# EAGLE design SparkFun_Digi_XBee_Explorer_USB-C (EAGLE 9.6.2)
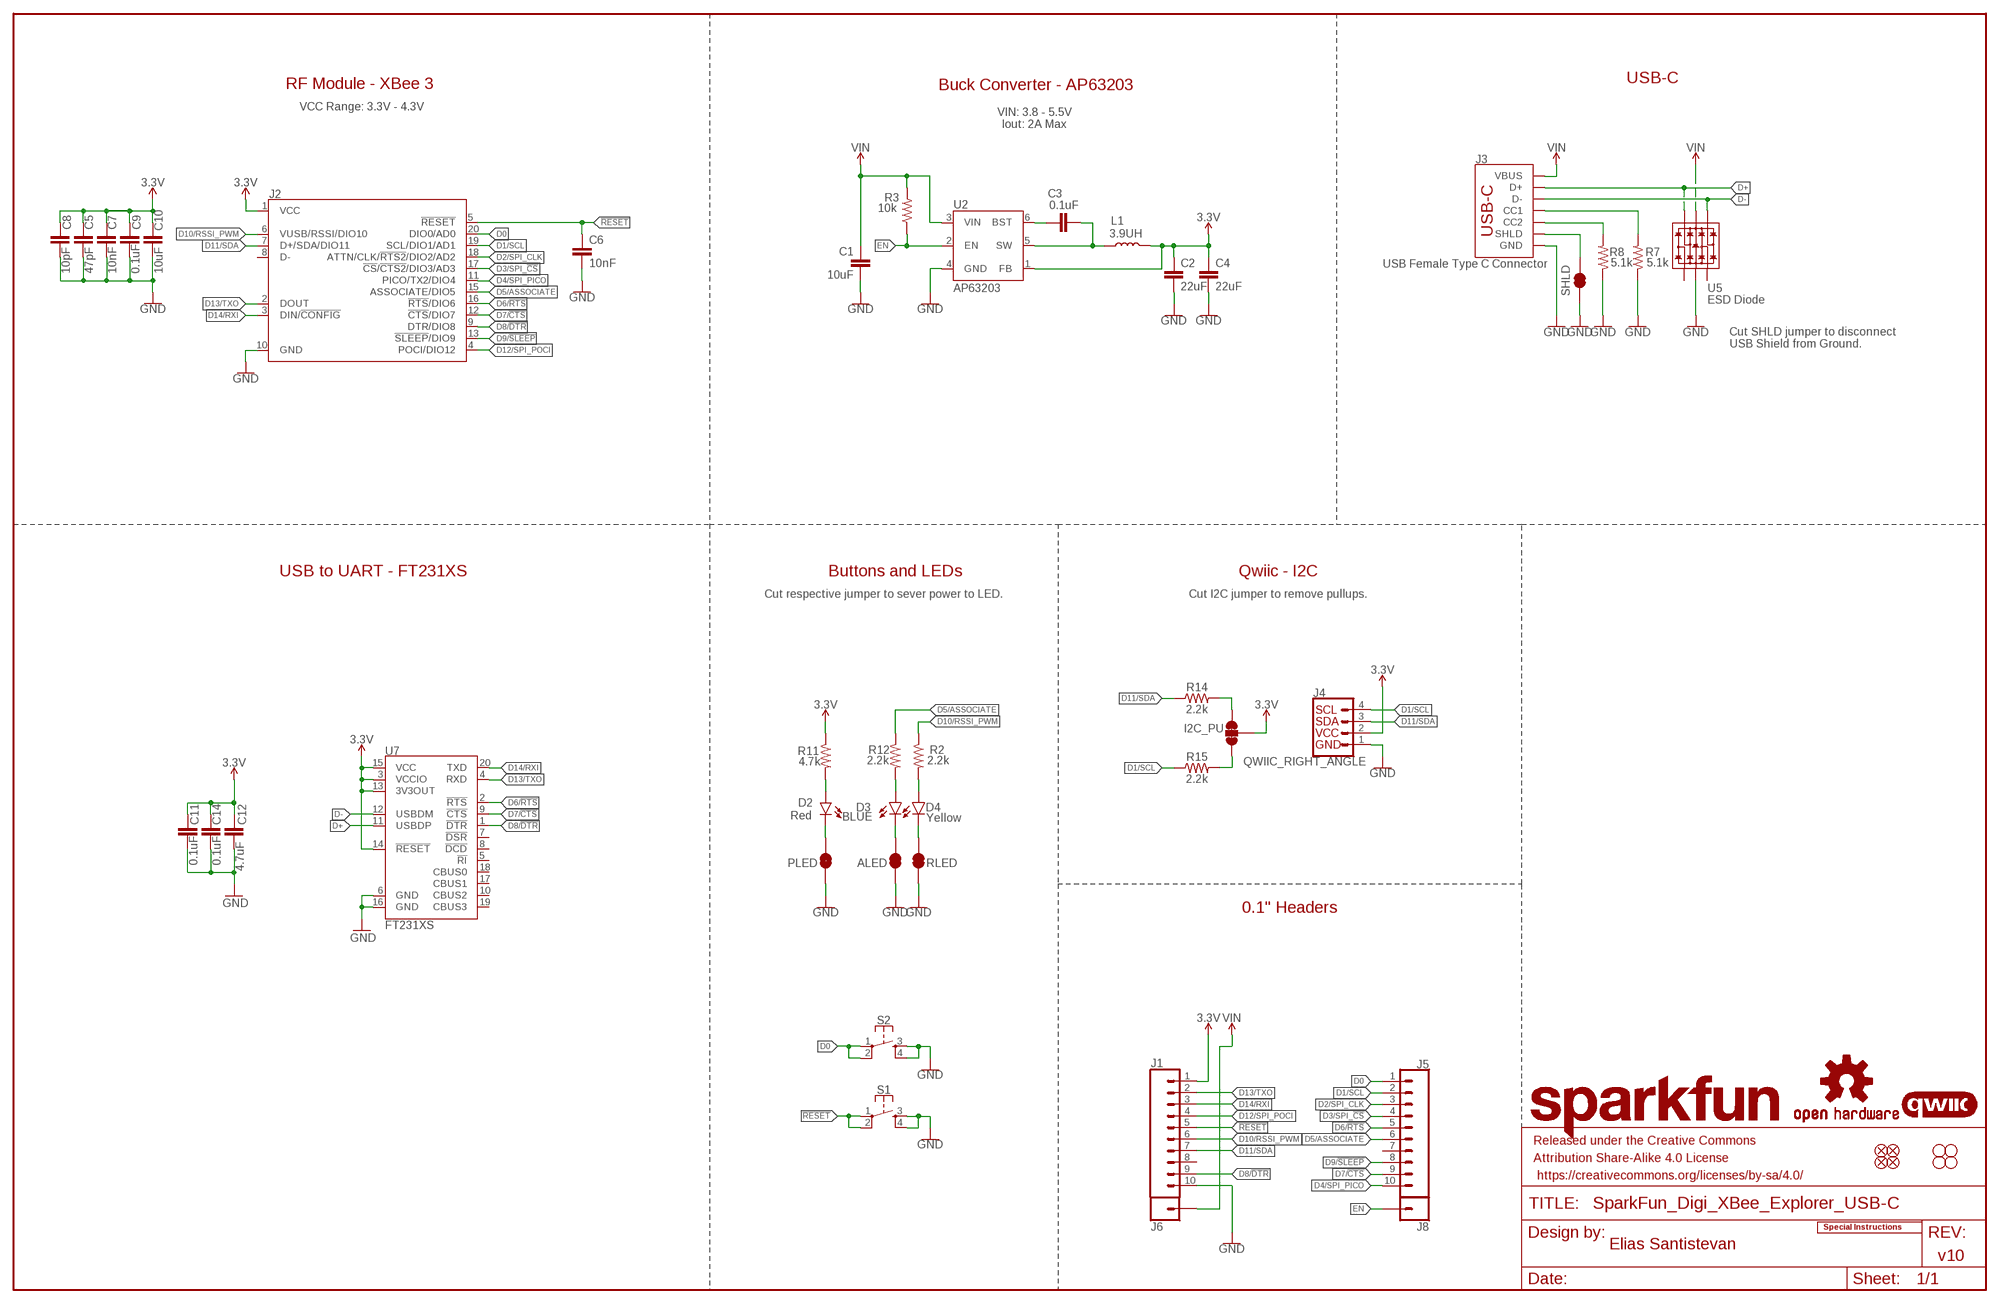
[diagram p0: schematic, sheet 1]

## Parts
ALED  JUMPER-SMT_2_NC_TRACE_SILK  [SMT-JUMPER_2_NC_TRACE_SILK]
C1  10uF  10UF-1210-50V-20%  [1210]
C2  22uF  22UF-0603-6.3V-20%  [0603]
C3  0.1uF  0.1UF-0603-25V-5%  [0603]
C4  22uF  22UF-0603-6.3V-20%  [0603]
C5  47pF  47PF-0603-50V-5%  [0603]
C6  10nF  10NF-0603-50V-10%  [0603]
C7  10nF  10NF-0603-50V-10%  [0603]
C8  10pF  10PF-0603-50V-5%  [0603]
C9  0.1uF  0.1UF-0603-25V-(+80/-20%)  [0603]
C10  10uF  10UF-0603-6.3V-20%  [0603]
C11  0.1uF  0.1UF-0603-25V-(+80/-20%)  [0603]
C12  4.7uF  4.7UF-0603-6.3V-(10%)  [0603]
C14  0.1uF  0.1UF-0603-25V-(+80/-20%)  [0603]
D2  Red  LED-RED_0603-KB  [LED-0603]
D3  BLUE  LED-BLUE0603  [LED-0603]
D4  Yellow  LED-YELLOW0603  [LED-0603]
FD1  FIDUCIAL1X2  [FIDUCIAL-1X2]
FD2  FIDUCIAL1X2  [FIDUCIAL-1X2]
FD3  FIDUCIAL1X2  [FIDUCIAL-1X2]
FD4  FIDUCIAL1X2  [FIDUCIAL-1X2]
FRAME1  FRAME-LEDGER  [CREATIVE_COMMONS]
H1  STAND-OFFTIGHT  [STAND-OFF-TIGHT]
H2  STAND-OFFTIGHT  [STAND-OFF-TIGHT]
H3  STAND-OFFTIGHT  [STAND-OFF-TIGHT]
H4  STAND-OFFTIGHT  [STAND-OFF-TIGHT]
I2C_PU  JUMPER-SMT_3_2-NC_TRACE_SILK  [SMT-JUMPER_3_2-NC_TRACE_SILK]
J1  CONN_01PTH_NO_SILK_STAND  [1X01_NO_SILK_STAND]
J2  XBEE_UPDATEXBEE_SMD  [XBEE3-SMD]
J3  USB Female Type C Connector  USB_C_4-LAYER-ISOLATED  [USB-C-16P-4LAYER-ISOLATED]
J4  QWIIC_RIGHT_ANGLE  QWIIC_CONNECTORJS-1MM  [JST04_1MM_RA]
J5  CONN_10NO_SILK_PTH_FEMALE  [1X10_NO_SILK]
J6  CONN_10NO_SILK_PTH_FEMALE  [1X10_NO_SILK]
J8  CONN_01PTH_NO_SILK_STAND  [1X01_NO_SILK_STAND]
L1  3.9UH  [INDUCTOR_3.9UH]
LOGO1  SFE_LOGO_NAME.2_INCH  [SFE_LOGO_NAME_.2]
LOGO2  OSHW-LOGOS  [OSHW-LOGO-S]
LOGO3  QWIIC_LOGO_4MM  [QWIIC_4MM]
LOGO4  SPECIAL_INSTRUCTIONS-ORDERING  [ORDERING_INSTRUCTIONS]
PLED  JUMPER-SMT_2_NC_TRACE_SILK  [SMT-JUMPER_2_NC_TRACE_SILK]
R2  2.2k  2.2KOHM-0603-1/10W-1%  [0603]
R3  10k  10KOHM-0603-1/10W-1%  [0603]
R7  5.1k  5.1KOHM5.1KOHM-0603-1/10W-1%  [0603]
R8  5.1k  5.1KOHM5.1KOHM-0603-1/10W-1%  [0603]
R11  4.7k  4.7KOHM-0603-1/10W-1%  [0603]
R12  2.2k  2.2KOHM-0603-1/10W-1%  [0603]
R14  2.2k  2.2KOHM-0603-1/10W-1%  [0603]
R15  2.2k  2.2KOHM-0603-1/10W-1%  [0603]
RLED  JUMPER-SMT_2_NC_TRACE_SILK  [SMT-JUMPER_2_NC_TRACE_SILK]
S1  MOMENTARY-SWITCH-SPST-2-SMD-5.2MM-TALL  [TACTILE_SWITCH_SMD_5.2MM]
S2  MOMENTARY-SWITCH-SPST-2-SMD-5.2MM-TALL  [TACTILE_SWITCH_SMD_5.2MM]
SHLD  JUMPER-SMT_2_NC_TRACE_SILK  [SMT-JUMPER_2_NC_TRACE_SILK]
U2  AP63203  [SOT23-6]
U5  ESD Diode  TVS_DIODE_ARRAY_DT1042-04SO-7  [SOT-23-6]
U7  FT231XS  [SSOP20_L]

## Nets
3.3V: C2.1 C4.1 C5.1 C7.1 C8.1 C9.1 C10.1 C11.1 C12.1 C14.1 I2C_PU.2 J2.1(VCC) J4.2 J6.1 L1.P$2 R11.1 U2.1(FB) U7.3(VCCIO) U7.13(3V3OUT) U7.14(!RESET) U7.15(VCC)
!RESET!: C6.1 J2.5(!RESET!) J6.5 S1.1 S1.2
D0: J2.20(DIO0/AD0) J5.1 S2.1 S2.2
D1/SCL: J2.19(SCL/DIO1/AD1) J4.4 J5.2 R15.1
D2/SPI_CLK: J2.18(ATTN/CLK/!RTS2!/DIO2/AD2) J5.3
D3/SPI_!CS!: J2.17(!CS!/!CTS2!/DIO3/AD3) J5.4
D4/SPI_PICO: J2.11(PICO/TX2/DIO4) J5.10
D5/ASSOCIATE: J2.15(ASSOCIATE/DIO5) J5.6 R12.1
D6/!RTS!: J2.16(!RTS!/DIO6) J5.5 U7.2(!RTS)
D7/!CTS!: J2.12(!CTS!/DIO7) J5.9 U7.9(!CTS)
D8/!DTR!: J2.9(DTR/DIO8) J6.9 U7.1(!DTR)
D9/!SLEEP!: J2.13(!SLEEP!/DIO9) J5.8
D10/RSSI_PWM: J2.6(VUSB/RSSI/DIO10) J6.6 R2.1
D11/SDA: J2.7(D+/SDA/DIO11) J4.3 J6.7 R14.1
D12/SPI_POCI: J2.4(POCI/DIO12) J6.4
D13/TXO: J2.2(DOUT) J6.2 U7.4(RXD)
D14/RXI: J2.3(DIN/!CONFIG!) J6.3 U7.20(TXD)
D+ [Diff pairs]: J3.A6(D+) J3.B6(D+) U5.6(IO4) U7.11(USBDP)
D- [Diff pairs]: J3.A7(D-) J3.B7(D-) U5.4(IO3) U7.12(USBDM)
EN: J8.1 R3.1 U2.2(EN)
GND: ALED.1 C1.2 C2.2 C4.2 C5.2 C6.2 C7.2 C8.2 C9.2 C10.2 C11.2 C12.2 C14.2 J2.10(GND) J3.GND J3.GND2(GND) J4.1 J6.10 PLED.1 R7.1 R8.1 RLED.1 S1.3 S1.4 S2.3 S2.4 SHLD.1 U2.4(GND) U5.2(VSS) U7.6(GND) U7.16(GND)
N$1: C3.1 U2.6(BST)
N$2: D4.A R2.2
N$3: D4.C RLED.2
N$5: J3.B5(CC2) R8.2
N$6: J3.A5(CC1) R7.2
N$7: D2.A R11.2
N$8: C3.2 L1.P$1 U2.5(SW)
N$11: I2C_PU.3 R14.2
N$12: D3.A R12.2
N$13: I2C_PU.1 R15.2
N$21: ALED.2 D3.C
N$23: D2.C PLED.2
SHLD: J3.SHLD1(SHLD) J3.SHLD2(SHLD) J3.SHLD3(SHLD) J3.SHLD4(SHLD) J3.SHLD5(SHLD) J3.SHLD6(SHLD) J3.SHLD7(SHLD) J3.SHLD8(SHLD) SHLD.2
VIN: C1.1 J1.1 J3.VBUS1(VBUS) J3.VBUS2(VBUS) R3.2 U2.3(VIN) U5.5(VCC)
Unconnected: J2.8(D-) J5.7 J6.8 U5.1(IO1) U5.3(IO2) U7.5(!RI) U7.7(!DSR) U7.8(!DCD) U7.10(CBUS2) U7.17(CBUS1) U7.18(CBUS0) U7.19(CBUS3)

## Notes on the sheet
- RF Module - XBee 3 | Buck Converter - AP63203 | USB-C
- VCC Range: 3.3V - 4.3V
- VIN: 3.8 - 5.5V
  Iout: 2A Max
- Cut SHLD jumper to disconnect
  USB Shield from Ground.
- USB to UART - FT231XS | Buttons and LEDs | Qwiic - I2C
- Cut respective jumper to sever power to LED. | Cut I2C jumper to remove pullups.
- 0.1" Headers
- Elias Santistevan
- v10

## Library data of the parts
ALED PLED RLED SHLD = SparkFun-Jumpers:JUMPER-SMT_2_NC_TRACE: Normally closed trace jumper
C1 = SparkFun-Capacitors:10UF: 10.0µF ceramic capacitors; PROD_ID: CAP-09824
C2 C4 = SparkFun-Capacitors:22UF: 22µF ceramic capacitors; PROD_ID: CAP-14464
C3 = SparkFun-Capacitors:0.1UF: 0.1µF ceramic capacitors; PROD_ID: CAP-08604
C5 = SparkFun-Capacitors:47PF: 47pF ceramic capacitors; PROD_ID: CAP-08913
C6 C7 = SparkFun-Capacitors:10NF: 0.01uF/10nF/10,000pF ceramic capacitors; PROD_ID: CAP-00867
C8 = SparkFun-Capacitors:10PF: 10pF ceramic capacitors; PROD_ID: CAP-11812
C9 C11 C14 = SparkFun-Capacitors:0.1UF: 0.1µF ceramic capacitors; PROD_ID: CAP-00810
C10 = SparkFun-Capacitors:10UF: 10.0µF ceramic capacitors; PROD_ID: CAP-11015
C12 = SparkFun-Capacitors:4.7UF: 4.7µF ceramic capacitors; PROD_ID: CAP-08280
D2 = SparkFun-LED:LED-RED: Red SMD LED; PROD_ID: DIO-17976
D3 = SparkFun-LED:LED-BLUE: Blue SMD LED; PROD_ID: DIO-08575
D4 = SparkFun-LED:LED-YELLOW: Yellow SMD LED; PROD_ID: DIO-09003
FD1-FD4 = SparkFun-Aesthetics:FIDUCIAL: Fiducial Alignment Points
FRAME1 = SparkFun-Aesthetics:FRAME-LEDGER: Schematic Frame - Ledger
H1-H4 = SparkFun-Hardware:STAND-OFF: Stand Off
I2C_PU = SparkFun-Jumpers:JUMPER-SMT_3_2-NC_TRACE: Normally closed trace jumper (2 of 2 connections) This jumper has a trace between all three pads so they are normally closed (NC). Use a razor knife to open the connection(s). For best results follow the IPC guidelines for cutting traces: Cutout at least 0.063 mm (0.005 in). Remove all loose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
J1 J8 = SparkFun-Connectors:CONN_01: Single connection point. Often used as Generic Header-pin footprint for 0.1 inch spaced/style header connections
J2 = xbee_smart_modem:XBEE_UPDATE: XBee 3 Cat 1 Smart Modem
J3 = SparkFun-Connectors:USB_C: USB Type C 16Pin Connector Super Speed pins not available on the 16-pin purely SMD connector so this part is best for USB 2.0 implementations. D1 and D2 are tied together enabling D+/- no matter which way the cable is plugged into the connector. The two channel configuration pins (CC1/2) are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; PROD_ID: CONN-14122
J4 = SparkFun-Connectors:QWIIC_CONNECTOR: SparkFun I2C Standard Qwiic Connector An SMD 1mm pitch JST connector makes it easy and quick (get it? Qwiic?) to connect I2C devices to each other. The Qwiic system enables fast and solderless connection between popular platforms and various sensors and actuators. We carry 200mm, 100mm, 50mm, and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; PROD_ID: CONN-13694
J5 J6 = SparkFun-Connectors:CONN_10: Multi connection point. Often used as Generic Header-pin footprint for 0.1 inch spaced/style header connections On any of the 0.1 inch spaced packages, you can populate with these: Break Away Headers - Straight (PRT-00116) Break Away Male Headers - Right Angle (PRT-00553) Female Headers (PRT-00115)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
L1 = SparkFun-Coils:3.9UH: Würth's Electronik 3.9uH Inductor; PROD_ID: NDUC-18014
LOGO1 = SparkFun-Aesthetics:SFE_LOGO_NAME: SparkFun Font Logo
LOGO2 = SparkFun-Aesthetics:OSHW-LOGO: Open-Source Hardware (OSHW) Logo
LOGO3 = SparkFun-Aesthetics:QWIIC_LOGO: Qwiic Logos for placement on schematic and PCB. The 5.5mm silk logo is best for placing next to Qwiic connector.
LOGO4 = SparkFun-Aesthetics:SPECIAL_INSTRUCTIONS: Special Ordering/Production Instructions Alert
R2 R12 R14 R15 = SparkFun-Resistors:2.2KOHM: 2.2kΩ resistor; PROD_ID: RES-08272
R3 = SparkFun-Resistors:10KOHM: 10kΩ resistor; PROD_ID: RES-00824
R7 R8 = SparkFun-Resistors:5.1KOHM; PROD_ID: RES-12083
R11 = SparkFun-Resistors:4.7KOHM: 4.7kΩ resistor; PROD_ID: RES-07857
S1 S2 = SparkFun-Switches:MOMENTARY-SWITCH-SPST-2: Momentary Switch (Pushbutton) - SPST - Two Circuits Normally-open (NO) SPST momentary switches (buttons, pushbuttons). Schematic symbol includes two switch circuits. Variants SMD-4.6MMX2.8MM - 4.60mm x 2.80mm Tactile Momentary Button Switch - Used on SparkFun Pro Micro - RP2040 SMD-5.2MM - Mini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; PROD_ID: SWCH-14139
U2 = SparkFun-IC-Power:AP63203: Diodes Inc. AP63203 3.8V-32V input 3.3V Buck The AP63200/AP63201/AP63203/AP63205 is a 2A, synchronous buck converter with a wide input voltage range of 3.8V to 32V and fully integrates a 125mΩ high-side power MOSFET and a 68mΩ lowside power MOSFET to provide high-efficiency step-down DC/DC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; PROD_ID: VREG-15244
U5 = SparkFun-DiscreteSemi:TVS_DIODE_ARRAY; PROD_ID: IC-13538
U7 = SparkFun-IC-Comms:FT231X: FTDI FT231X Full Speed USB to Full-handshake UART This USB2.0 Full Speed IC offers a compact bridge to full handshake UART interfaces. The device is a UART, capable of operating up to 3MBaud, with low power consumption (8mA). The FT231X includes the complete FT-X series feature set and enables USB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; PROD_ID: IC-11524

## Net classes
1 POWER: width 0.559 mm, drill 0.305 mm
2 Diff pairs: width 0.203 mm, drill 0.305 mm, clearance 0.152 mm

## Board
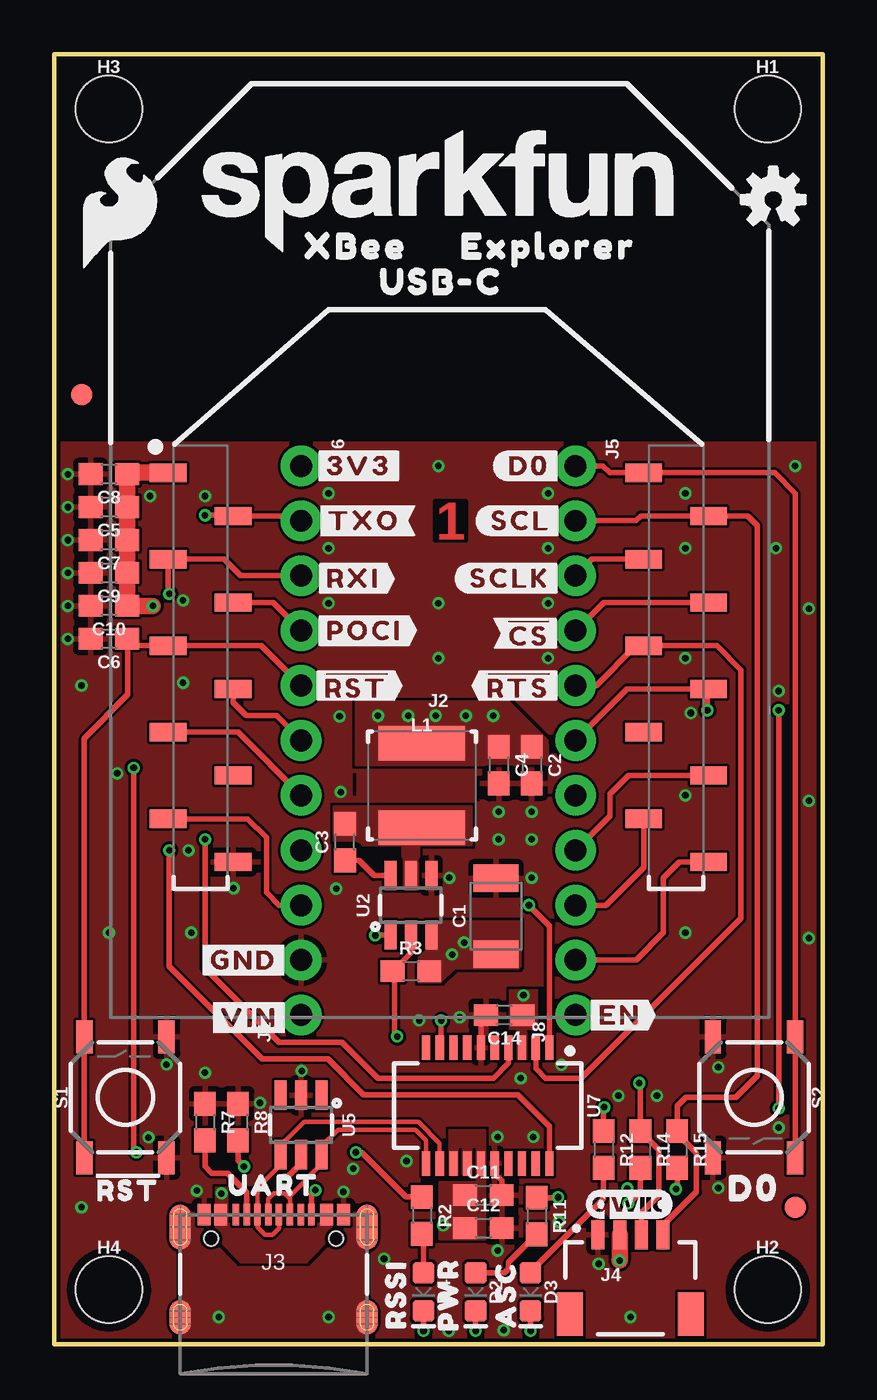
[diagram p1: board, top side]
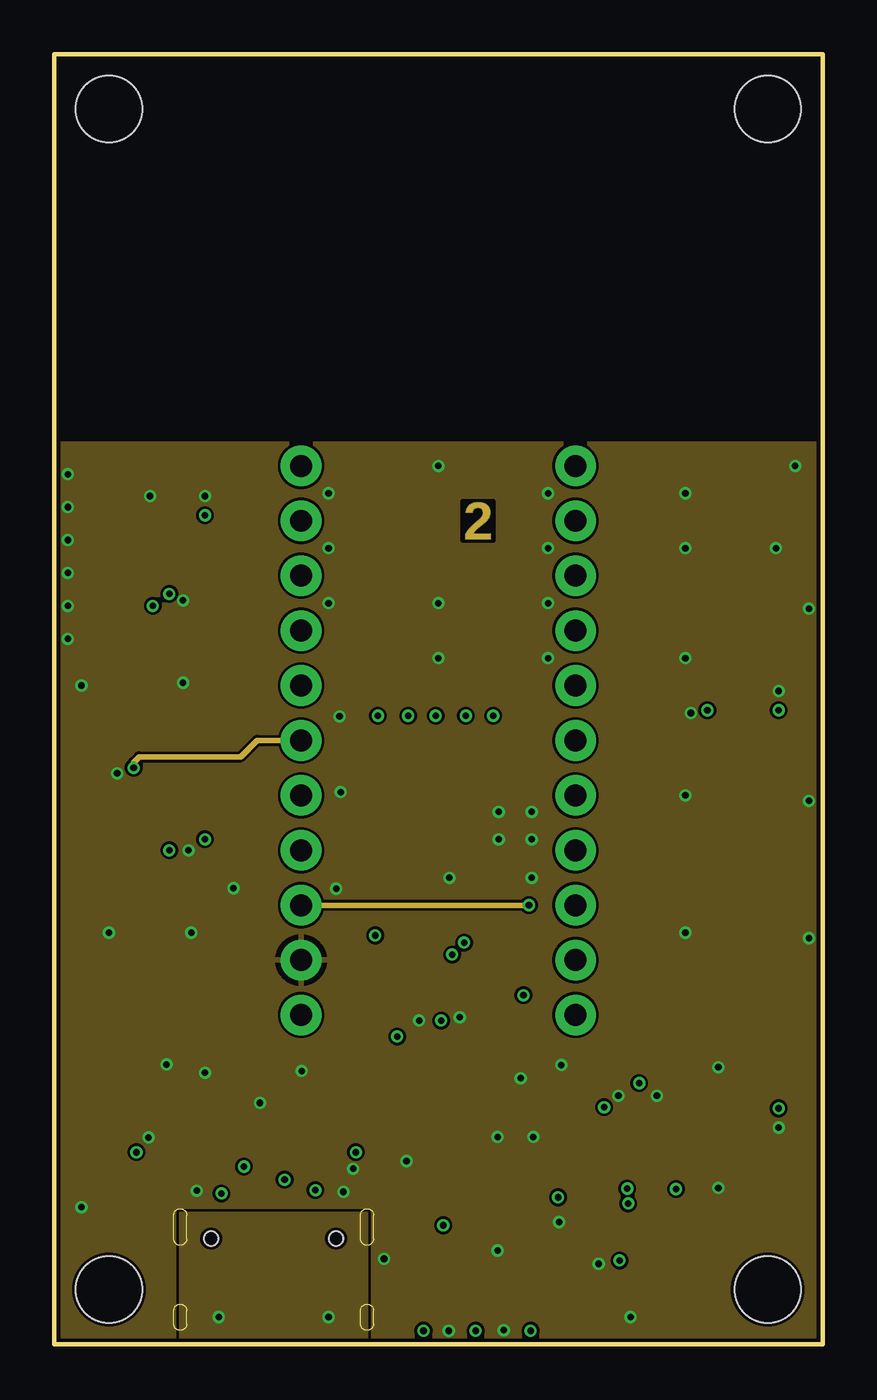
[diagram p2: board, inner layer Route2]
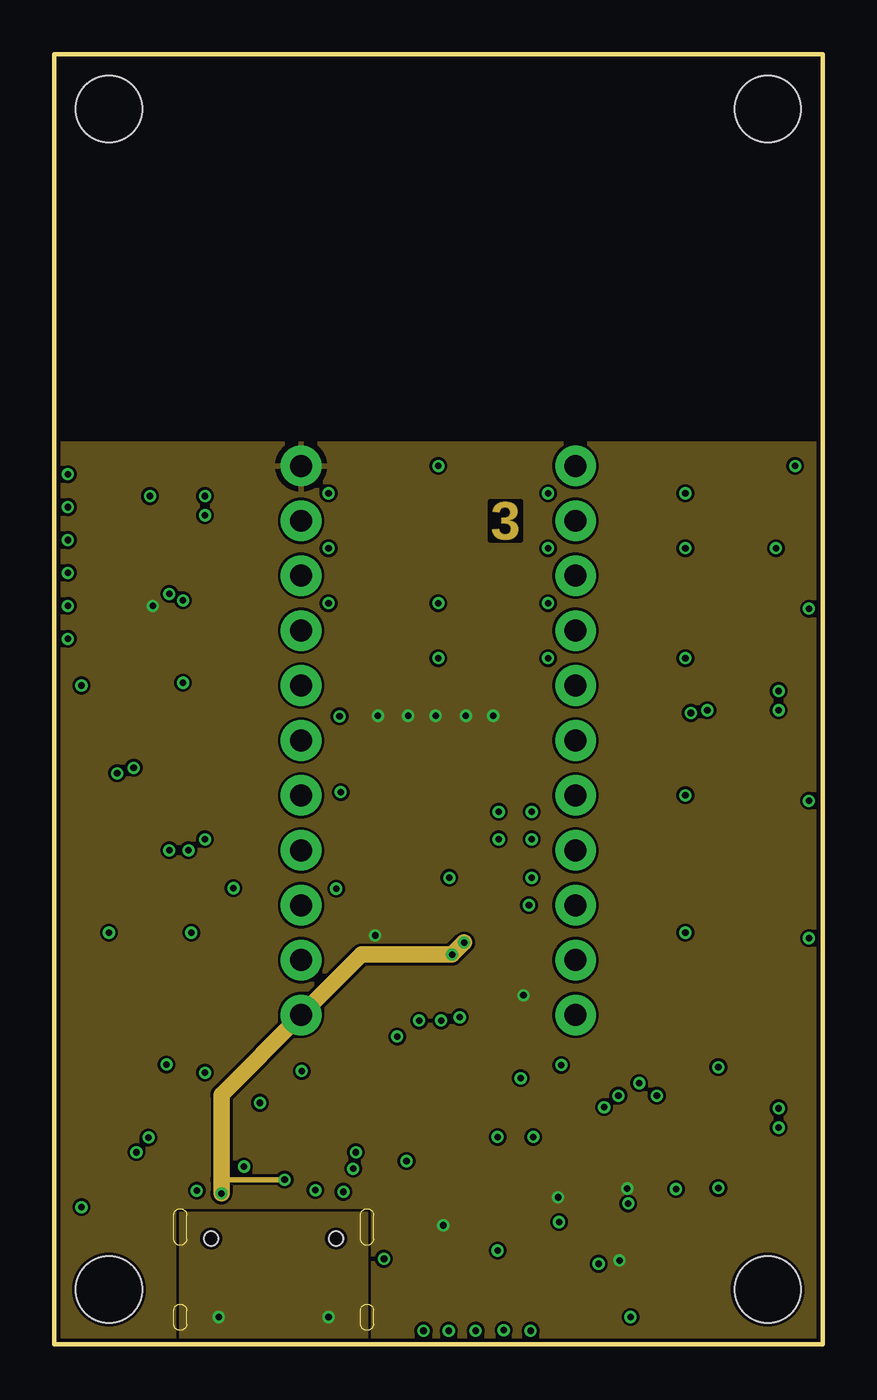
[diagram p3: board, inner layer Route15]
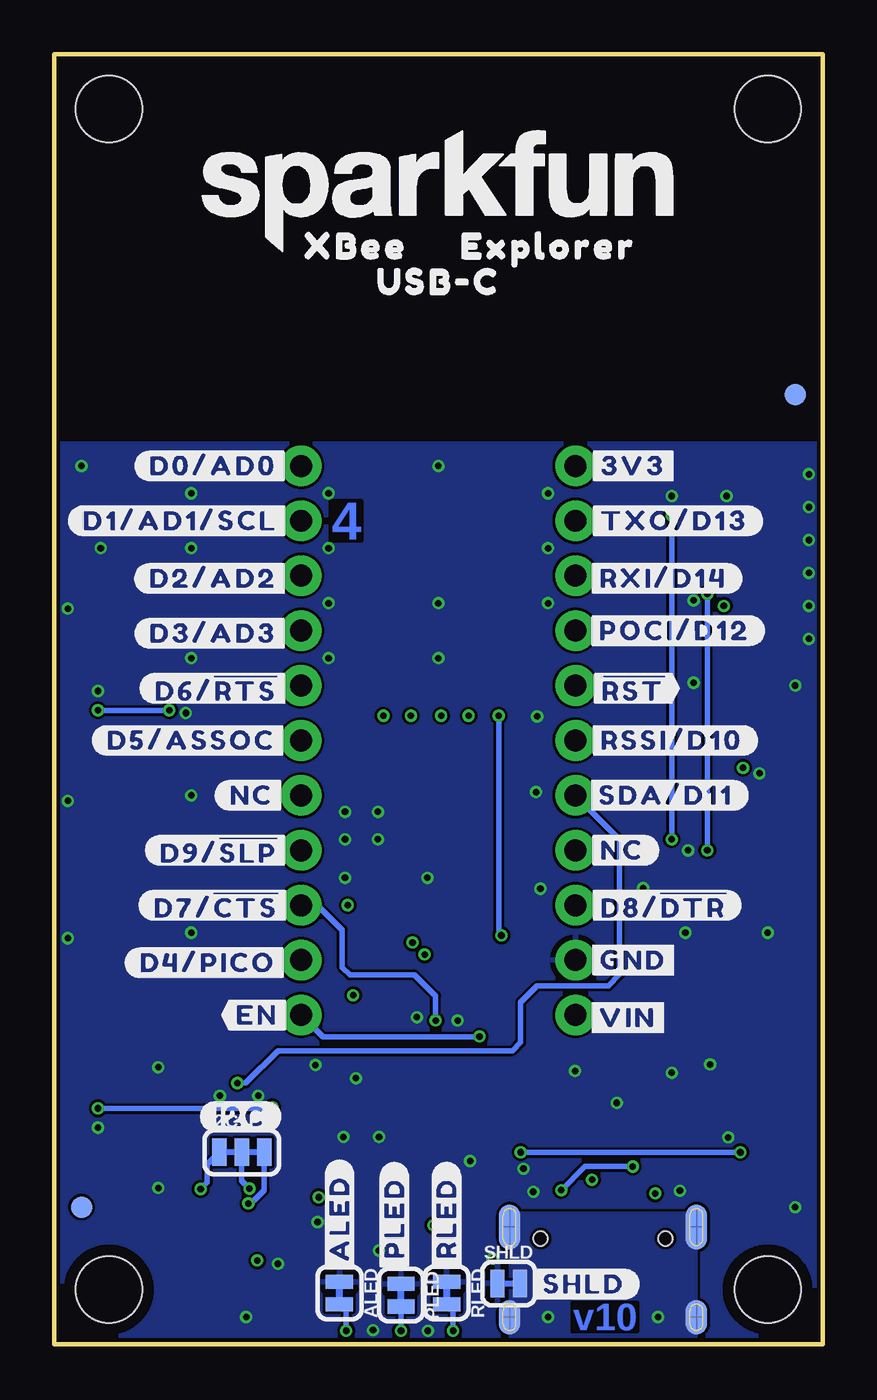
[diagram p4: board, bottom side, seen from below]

Size 35.56 x 59.69 mm. Coordinates in mm from the lower left corner, seen from the top.
Outline: 0,59.69 0,0 35.56,0 35.56,59.69 0,59.69
Copper layers (1*2*15*16): Top 0.035559375mm / dielectric 0.47751875mm / Route2 0.035559375mm / dielectric 0.47751875mm / Route15 0.035559375mm / dielectric 0.47751875mm / Bottom 0.035559375mm
Design rules "SparkFun-4-Layer-Minimum-JLCPCB": minimum track width 5mil, minimum drill 0.2mm, track to track 5mil, track to pad 5mil, pad to pad 5mil, via to via 5mil, smd to smd 5mil, copper to edge 7mil, drill to drill 7mil, minimum pad ring 5mil, minimum via ring 5mil, stop-mask expansion 2.5mil, vias tented up to drill 25mil, thermal gap 10mil
tRestrict: area 13.8,25.4 to 14,26.4; area 19.6,25.1 to 19.7,26.3

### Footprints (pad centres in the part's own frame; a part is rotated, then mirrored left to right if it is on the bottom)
SMT-JUMPER_2_NC_TRACE_SILK = smd 0.66 x 1.27: 1 -0.521,0; 2 0.521,0
1210 = smd 1.27 x 2.06: 1 -1.755,0; 2 1.755,0
0603 = smd 1.1 x 1: 1 -0.85,0; 2 0.85,0
LED-0603 = smd 1 x 1: A -0.877,0; C 0.877,0
FIDUCIAL-1X2 = smd 1 x 1: 1 0,0
STAND-OFF-TIGHT = hole 3.048: 0,0
SMT-JUMPER_3_2-NC_TRACE_SILK = smd 0.66 x 1.27: 1 -1.041,0; 2 0,0; 3 1.041,0
1X01_NO_SILK_STAND = drill 1.016 pad 1.88: 1 0,0
XBEE3-SMD = smd 1.7 x 0.85: 1 -12.5,11.11; 2 -9.5,9.11; 3 -12.5,7.11; 4 -9.5,5.11; 5 -12.5,3.11; 6 -9.5,1.11; 7 -12.5,-0.89; 8 -9.5,-2.89; 9 -12.5,-4.89; 10 -9.5,-6.89; 11 12.5,-6.89; 12 9.5,-4.89; 13 12.5,-2.89; 14 9.5,-0.89; 15 12.5,1.11; 16 9.5,3.11; 17 12.5,5.11; 18 9.5,7.11; 19 12.5,9.11; 20 9.5,11.11
USB-C-16P-4LAYER-ISOLATED = smd 0.3 x 1: A5 -1.25,-0.34; A6 -0.25,-0.34; A7 0.25,-0.34; A8 1.25,-0.34; B5 1.75,-0.34; B6 0.75,-0.34; B7 -0.75,-0.34; B8 -1.75,-0.34 | smd 0.6 x 1: GND -3.225,-0.34; GND2 3.225,-0.34; VBUS1 -2.45,-0.34; VBUS2 2.45,-0.34 | smd 1 x 2.1: SHLD1 -4.32,-0.915; SHLD2 4.32,-0.915 | smd 1 x 2.1 bottom: SHLD3 -4.32,-0.915; SHLD4 4.32,-0.915 | smd 1 x 1.6: SHLD5 -4.32,-5.095; SHLD8 4.32,-5.095 | smd 1 x 1.6 bottom: SHLD6 -4.32,-5.095; SHLD7 4.32,-5.095 | hole 0.65: -2.89,-1.445; 2.89,-1.445
JST04_1MM_RA = smd 0.6 x 1.35: 1 -1.5,0; 2 -0.5,0; 3 0.5,0; 4 1.5,0 | smd 1.2 x 2: NC1 2.8,-3.675; NC2 -2.8,-3.675
1X10_NO_SILK = drill 1.016 pad 1.88: 1 0,0; 2 2.54,0; 3 5.08,0; 4 7.62,0; 5 10.16,0; 6 12.7,0; 7 15.24,0; 8 17.78,0; 9 20.32,0; 10 22.86,0
INDUCTOR_3.9UH = smd 4 x 1.6: P$1 0,-2; P$2 0,1.9
TACTILE_SWITCH_SMD_5.2MM = smd 1.524 x 0.762: 1 -2.794,1.905; 2 2.794,1.905; 3 -2.794,-1.905; 4 2.794,-1.905
SOT23-6 = smd 0.55 x 1.35: 1 -0.95,-1.375; 2 0,-1.375; 3 0.95,-1.375; 4 0.95,1.375; 5 0,1.375; 6 -0.95,1.375
SOT-23-6 = smd 0.55 x 1.35: 1 -0.95,-1.375; 2 0,-1.375; 3 0.95,-1.375; 4 0.95,1.375; 5 0,1.375; 6 -0.95,1.375
SSOP20_L = smd 0.381 x 1.143: 1 -2.857,-2.68; 2 -2.223,-2.68; 3 -1.587,-2.68; 4 -0.953,-2.68; 5 -0.318,-2.68; 6 0.318,-2.68; 7 0.953,-2.68; 8 1.587,-2.68; 9 2.223,-2.68; 10 2.857,-2.68; 11 2.857,2.68; 12 2.223,2.68; 13 1.587,2.68; 14 0.953,2.68; 15 0.318,2.68; 16 -0.318,2.68; 17 -0.953,2.68; 18 -1.587,2.68; 19 -2.223,2.68; 20 -2.857,2.68

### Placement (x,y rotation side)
ALED  22.35,2.38 270 bottom
C1  20.45,19.81 90 top
C2  22.1,26.8 270 top
C3  13.46,23.24 90 top
C4  20.57,26.8 270 top
C5  2.54,38.73 180 top
C6  2.54,32.64 180 top
C7  2.54,37.21 180 top
C8  2.54,40.26 180 top
C9  2.54,35.69 180 top
C10  2.54,34.16 180 top
C11  19.86,6.91 0 top
C12  19.86,5.38 0 top
C14  20.83,15.24 180 top
D2  19.51,2.44 270 top
D3  22.05,2.44 270 top
D4  17.09,2.44 270 top
FD1  1.27,43.94 0 top
FD2  1.27,43.94 0 bottom
FD3  34.29,6.35 0 top
FD4  34.29,6.35 0 bottom
FRAME1  not placed on the board
H1  33.02,57.15 0 top
H2  33.02,2.54 0 top
H3  2.54,57.15 0 top
H4  2.54,2.54 0 top
I2C_PU  26.87,8.89 0 bottom
J1  11.43,15.24 90 top
J2  17.78,29.21 0 top
J3  10.16,6.35 0 top
J4  26.67,5.08 0 top
J5  24.13,40.64 270 top
J6  11.43,40.64 270 top
J8  24.13,15.24 90 top
L1  17.02,25.91 0 top
LOGO1  17.78,53.34 0 top
LOGO2  33.27,52.96 0 top
LOGO3  26.62,6.48 0 top
LOGO4  not placed on the board
PLED  19.51,2.28 270 bottom
R2  17.02,5.97 270 top
R3  16.51,17.27 0 top
R7  6.99,10.29 270 top
R8  8.51,10.29 270 top
R11  22.33,5.94 270 top
R12  25.43,9.02 270 top
R14  27.13,9.02 270 top
R15  28.83,9.02 270 top
RLED  17.4,2.38 270 bottom
S1  3.3,11.43 90 top
S2  32.38,11.43 270 top
SHLD  14.53,2.82 0 bottom
U2  16.51,20.32 0 top
U5  11.43,10.16 180 top
U7  20.07,11.05 180 top
U$1  [RSSI31]  15.82,2.31 90 top
U$2  [PWR29]  18.24,2.31 90 top
U$3  [#GND#0]  8.76,17.78 0 top
U$4  [#SHLD#36]  11.05,2.79 0 bottom
U$5  [#NC#1]  9.27,22.86 0 bottom
U$6  [#D3#AD3#23]  28.19,32.89 0 bottom
U$7  [#NC#3]  26.42,25.4 0 bottom
U$8  [#D0#AD0#18]  28.19,40.64 0 bottom
U$9  [#3V3#1]  14.1,40.64 0 top
U$10  [XBEE340]  13.97,50.8 0 top
U$11  [#D1#AD1#SCL#8]  29.72,38.1 0 bottom
U$12  [#GND#0]  8.76,17.78 0 bottom
U$13  [#D8##DTR##27]  7.37,20.32 0 bottom
U$14  [#RSSI#D10#17]  6.99,27.94 0 bottom
U$15  [#SDA#D11#9]  7.24,25.4 0 bottom
U$16  [##RST##15]  8.76,30.35 0 bottom
U$17  [#POCI#D12#24]  6.86,33.02 0 bottom
U$18  [#RXI#D14#15]  7.37,35.43 0 bottom
U$19  [#D2#AD2#19]  28.19,35.43 0 bottom
U$20  [#D6##RTS##25]  28.07,30.35 0 bottom
U$21  [#TXO#8]  14.35,38.1 0 top
U$22  [#TXO#D13#13]  6.86,38.1 0 bottom
U$23  [XBEE340]  21.59,50.8 0 bottom
U$24  [USB#C1342]  17.91,49.15 0 top
U$25  [USB#C1342]  17.78,49.15 0 bottom
U$26  [#I2C#33]  26.92,10.54 0 bottom
U$27  [#RXI#7]  13.84,35.43 0 top
U$28  [UART34]  10.16,7.37 0 top
U$29  [ASC32]  20.9,2.31 90 top
U$30  [#RST#30]  3.43,7.25 0 top
U$31  [EXPLORER1344]  22.86,50.8 0 top
U$32  [EXPLORER1344]  12.7,50.8 0 bottom
U$35  [#D5#ASSOC#25]  29.21,27.94 0 bottom
U$36  [#D9##SLP##28]  27.94,22.86 0 bottom
U$37  [#D7##CTS##26]  28.07,20.32 0 bottom
U$38  [#D4#PICO#25]  28.45,17.65 0 bottom
U$40  [D03]  32.38,7.23 0 top
U$44  [#3V3#1]  8.76,40.64 0 bottom
U$45  [#POCI#32]  14.35,33.02 0 top
U$46  [#VIN#4]  9.02,15.11 0 bottom
U$48  [#EN#17]  26.16,15.24 0 top
U$49  [#ALED#21]  22.35,5.84 90 bottom
U$51  [#RLED#22]  17.4,5.84 90 bottom
U$52  [#PLED#20]  19.81,5.84 90 bottom
U$54  [##RST##13]  13.97,30.48 0 top
U$58  [##RTS##14]  21.46,30.48 0 top
U$59  [##CS##26]  21.97,32.89 0 top
U$60  [#SCLK#33]  21.08,35.43 0 top
U$61  [SFE_LOGO_FLAME_.2]  3.05,52.32 0 top
U$63  [SFE_LOGO_NAME_.2]  17.78,53.34 0 bottom
U$64  [#SCL#9]  21.59,38.1 0 top
U$65  [#D0#3]  21.97,40.64 0 top
U$66  [#VIN#4]  9.02,15.11 0 top
U$67  [#EN#15]  26.16,15.24 0 bottom

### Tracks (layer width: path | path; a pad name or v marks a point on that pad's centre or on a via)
3.3V  (via drill 0.3)
  Top 0.254: U2.1 14.86,18.95 v14.86,18.92 | v23.32,6.81 23.3,6.79 R11.1
  Top 0.762: J2.1 3.45,40.32 C8.1 C5.1 C7.1 C9.1 C10.1 v4.57,34.16 | J4.2 v26.17,3.89 v26.16,3.89
  Bottom 0.254: v14.86,18.92 14.99,19.05 v14.99,29.08 | I2C_PU.2 26.87,7.57 v26.52,7.21
  other vias: 17.65,29.08 16.38,29.08 19.05,29.08 18.01,5.51 21.72,16.15 20.32,29.08
  pour Route15 (isolate 0.127, rank 3): 0,0 35.56,0 35.56,41.66 0,41.66
  pour Top (isolate 0.305, no thermals): 13.97,26.8 22.86,26.8 22.86,27.94 21.06,29.74 13.97,29.74
  pour Top (no thermals): 17.83,7.49 17.83,4.88 19.94,4.88 19.94,9.91 18.29,9.91 18.29,7.87 18.67,7.87 18.67,9.14 18.92,9.14 18.92,7.87 19.3,7.87 19.3,9.14 19.56,9.14 19.56,7.49
  pour Top (no thermals): 21.84,13.21 21.84,14.61 22.35,14.61 22.35,16.38 21.08,16.38 21.08,14.61 21.46,14.61 21.46,13.21
!RESET!
  Top 0.254: J6.5 9.59,32.32 J2.5 3.71,32.32 3.41,32.62 | 3.41,32.62 C6.1 | S1.1 S1.2 1.4,28.04 3.41,30.05 3.41,32.62
D0
  Top 0.254: J5.1 25.4,40.64 25.72,40.32 J2.20 33.34,40.32 34.29,39.37 S2.1 S2.2
D1/SCL
  Top 0.254: J5.2 26.92,38.1 27.14,38.32 J2.19 32.09,38.32 32.54,37.87 32.54,12.42 31.55,11.43 29.22,11.43 28.83,11.04 R15.1 28.83,9.75 29.72,8.87 29.72,7.06 28.17,5.51 J4.4
D2/SPI_CLK
  Top 0.254: J2.18 24.89,36.32 J5.3
D3/SPI_!CS!
  Top 0.254: J5.4 25.43,34.32 J2.17
D4/SPI_PICO
  Top 0.254: J5.10 24.14,17.79 26.94,17.79 28.19,19.05 28.19,21.59 28.92,22.32 J2.11
D5/ASSOCIATE  (via drill 0.3)
  Top 0.254: J5.6 26.51,30.32 J2.15 30.23,30.27 v30.23,29.34 | v25.45,10.97 25.43,10.95 R12.1 | v33.53,29.34 v33.53,10.92
  Bottom 0.254: v33.53,29.34 v30.23,29.34 | v33.53,10.92 25.5,10.92 v25.45,10.97
D6/!RTS!
  Top 0.254: J5.5 25.08,30.48 26.92,32.32 J2.16 30.66,32.32 31.77,31.21 31.77,19.71 24.38,12.32 22.73,12.32 22.29,12.76 U7.2
D7/!CTS!  (via drill 0.3)
  Top 0.254: J2.12 27.28,22.07 25.53,20.32 J5.9 | U7.9 17.91,13.79 v17.91,14.99
  Bottom 0.254: v17.91,14.99 17.91,16.13 18.87,17.09 21.87,17.09 22.23,17.45 22.23,19.18 23.36,20.32 J5.9
D8/!DTR!  (via drill 0.3)
  Top 0.254: J6.9 10.41,20.32 9.83,20.9 9.83,23.44 8.95,24.32 J2.9 | U7.1 22.92,19.37 v21.97,20.32
  Route2 0.254: v21.97,20.32 J6.9
D9/!SLEEP!
  Top 0.254: J5.8 25.72,24.45 25.72,25.46 26.57,26.32 J2.13
D10/RSSI_PWM  (via drill 0.3)
  Top 0.254: J2.6 8.28,29.69 8.89,29.08 10.29,29.08 J6.6 | R2.1 16.3,6.82 14.22,8.89 v13.97,8.89 | v3.68,26.67 3.68,9.02 v3.81,8.89
  Route2 0.254: v3.68,26.67 3.68,26.92 3.94,27.18 8.64,27.18 9.4,27.94 J6.6
  Bottom 0.254: v13.97,8.89 v3.81,8.89
D11/SDA  (via drill 0.3)
  Top 0.254: J2.7 8.51,28.32 J6.7 | v27.08,12.09 27.13,12.04 R14.1 27.99,9 27.99,6.91 27.17,6.09 J4.3
  Bottom 0.254: v27.08,12.09 26.7,12.09 25.2,13.59 14.35,13.59 13.97,13.97 13.97,15.82 13.21,16.59 9.92,16.59 9.4,17.11 9.4,23.37 J6.7
D12/SPI_POCI
  Top 0.254: J2.4 10.13,34.32 J6.4
D13/TXO  (via drill 0.3)
  Top 0.254: J6.2 11.21,38.32 J2.2 8.25,38.35 v6.99,38.35 | U7.4 21.02,13.02 20.32,12.32 14.99,12.32 13.34,13.97 10.41,13.97 6.99,17.4 v6.99,23.37
  Bottom 0.254: v6.99,23.37 v6.99,38.35
D14/RXI  (via drill 0.3)
  Top 0.254: J6.3 8.63,35.56 7.87,36.32 J2.3 5.28,34.78 v5.33,34.72 | U7.20 22.92,10.1 21.46,11.56 14.32,11.56 12.67,13.21 9.62,13.21 5.33,17.5 v5.33,22.86
  Bottom 0.254: v5.33,22.86 v5.33,34.72
D+
  Top 0.203: U7.11 17.21,9.44 16.71,9.93 13.13,9.93 12.32,9.12 12.32,9.02 12.32,8.85 | 12.32,8.85 U5.6 | J3.A6 9.91,6.74 10.16,6.99 10.67,6.99 10.85,6.81 | J3.B6 10.91,6.74 10.85,6.81 | 10.85,6.81 12.32,8.28 12.32,8.85
D-
  Top 0.203: J3.A7 10.41,5.38 10.11,5.08 9.75,5.08 9.41,5.42 J3.B7 9.41,7.25 10.48,8.32 U5.4 10.48,9.21 11.56,10.29 16.87,10.29 17.84,9.31 U7.12
EN  (via drill 0.3)
  Top 0.254: U2.2 16.51,18.12 R3.1 15.75,17.18 15.75,14.38 v15.88,14.25
  Bottom 0.254: J8.1 23.11,14.22 15.88,14.22 v15.88,14.25
GND  (via drill 0.3)
  Top 0.254: U7.6 19.75,15.24 C14.2 | U7.16 20.38,7.9 20.71,7.57 C11.2
  other vias: 20.57,24.64 22.1,24.64 18.29,21.59 20.57,23.37 22.1,23.37 0.64,40.26 0.64,38.73 0.64,37.21 0.64,35.69 0.64,34.16 0.64,32.64 33.53,30.23 29.46,29.21 22.1,21.59 16.89,14.99 13.84,8.13 4.37,9.58 5.21,12.95 30.73,12.83 30.73,7.24 25.2,3.73 6.99,39.24 5.97,34.42 6.22,22.86 2.92,26.42 11.46,12.65 6.99,12.57 9.53,11.18 17.78,40.64 34.29,40.64 26.67,1.27 1.27,6.35 13.26,25.55 13.21,29.06 8.31,21.11 13.06,21.08 20.52,9.6 18.77,15.14 13.39,7.06 20.8,0.66 18.26,0.64 15.27,3.96 33.53,10.03 5.97,30.61 29.21,39.37 29.21,36.83 29.21,31.75 29.21,25.4 29.21,19.05 6.35,19.05 2.54,19.05 4.45,39.24 33.4,36.83 23.47,12.93 22.86,36.83 22.86,34.29 22.86,31.75 17.78,31.75 17.78,34.29 12.7,34.29 12.7,36.83 12.7,39.37 22.86,39.37 1.27,30.48 34.92,25.15 34.92,18.8 34.92,34.04 21.59,12.32 6.6,7.11 26.11,11.51 22.17,9.6 20.52,4.34 16.31,8.48 23.37,5.66 27.89,11.51
  pour Bottom (isolate 0.127, rank 3): 0,0 35.56,0 35.56,41.66 0,41.66
  pour Route2 (isolate 0.127, rank 3): 0,0 35.56,0 35.56,41.66 0,41.66
  pour Top (rank 3): 0,41.66 35.56,41.66 35.56,0 0,0
N$1
  Top 0.254: U2.6 14.8,21.7 14.1,22.39 C3.1
N$2
  Top 0.254: R2.2 17.02,5.04 17.09,4.97 D4.A
N$3  (via drill 0.3)
  Top 0.254: D4.C v17.09,0.64
  Bottom 0.254: v17.09,0.64 D4.C RLED.2
N$5  (via drill 0.3)
  Top 0.254: J3.B5 11.91,6.96 v12.09,7.14 | v8.79,8.23 8.51,8.51 R8.2
  Bottom 0.254: v12.09,7.14 11,8.23 v8.79,8.23
N$6
  Top 0.254: J3.A5 8.91,7.04 8.03,7.92 7.29,7.92 6.99,8.23 R7.2
N$7
  Top 0.254: D2.A 20.84,3.31 21.03,3.5 21.03,3.8 R11.2
N$8
  pour Top (isolate 0.305, no thermals): 16.89,21.08 16.89,23.11 19.3,23.11 19.3,24.89 12.95,24.89 12.95,23.11 16.13,23.11 16.13,21.08
N$11  (via drill 0.3)
  Top 0.254: v26.57,6.53 26.72,6.68 26.74,6.68 27.13,7.07 R14.2
  Bottom 0.254: v26.57,6.53 26.42,6.68 26.3,6.68 25.83,7.14 I2C_PU.3
N$12
  Top 0.254: D3.A 22.05,3.37 25.43,6.74 R12.2
N$13  (via drill 0.3)
  Top 0.254: v28.78,7.19 28.83,7.24 R15.2
  Bottom 0.254: I2C_PU.1 28.47,8.33 28.47,7.49 v28.78,7.19
N$21  (via drill 0.3)
  Top 0.254: D3.C v22.05,0.64
  Bottom 0.254: ALED.2 D3.C v22.05,0.64
N$23  (via drill 0.3)
  Top 0.254: v19.51,0.64 D2.C
  Bottom 0.254: v19.51,0.64 PLED.2
SHLD  (via drill 0.3)
  other vias: 7.62,1.27 12.7,1.27
  pour Top (rank 2, no thermals): 5.84,0.25 5.84,6.1 14.48,6.1 14.48,0.25
  pour Bottom (rank 2, no thermals): 5.84,0.25 5.84,6.1 14.48,6.1 14.48,0.25
  pour Route15 (rank 2, no thermals): 5.84,0.25 5.84,6.1 14.48,6.1 14.48,0.25
  pour Route2 (rank 2, no thermals): 5.84,0.25 5.84,6.1 14.48,6.1 14.48,0.25
VIN  (via drill 0.3)
  Top 0.254: U5.5 11.43,8.38 v10.67,7.62
  Route15 0.254: v10.67,7.62 7.75,7.62
  Route15 0.762: v7.75,6.99 7.75,7.62 7.75,11.56 J1.1 14.22,18.03 v18.41,18.03 v18.97,18.59
  pour Top (no thermals): 16.89,16.76 16.89,17.91 17.27,18.29 17.27,19.56 21.59,19.56 21.59,17.5 21.49,17.4 18.54,17.4 17.91,16.76
  pour Top (no thermals): 7.49,7.24 7.49,4.95 8.64,3.81 11.68,3.81 12.83,4.95 12.83,6.48 12.45,6.48 12.45,5.71 12.32,5.59 8,5.59 8,7.24

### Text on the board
Top: 1
Route2: 2
Route15: 3
Bottom: 4 | v10
Measures: Units in Inches
tDocu: Four Layer Board | 1.6mm Thickness | Lead Free HASL | Elias Santistevan

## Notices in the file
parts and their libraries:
SparkFun-Capacitors: Licensing: Creative Commons ShareAlike 4.0 International - https://creativecommons.org/licenses/by-sa/4.0
SparkFun-Aesthetics: Released under the Creative Commons Attribution Share-Alike 4.0 License
SparkFun-Aesthetics: https://creativecommons.org/licenses/by-sa/4.0
